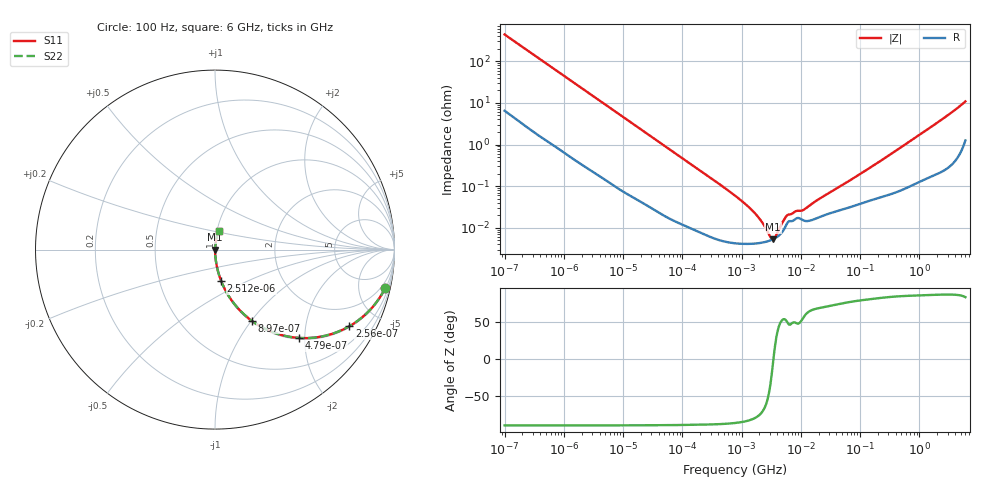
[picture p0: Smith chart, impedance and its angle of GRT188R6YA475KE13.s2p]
!Murata Part Number: GRT188R6YA475KE13
!These Parameters are Measured in Series Mode Connection
!Data Generated on Jun 19, 2026
!  o--ll--o
!Port1  Port2
!  o------o
!Operation Temp=25[degC], DC Bias Voltage=0[V]
!Freq. Start=100[Hz] Stop=6[GHz] 401[Steps]
# Hz S RI R 50
!Freq.(Hz) S11(Real) S11(Imag) S21(Real) S21(Imag) S12(Real) S12(Imag) S22(Real) S22(Imag)
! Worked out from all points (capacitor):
!   401 points, 100 Hz to 6 GHz, reference 50 ohm
!   read as one part in series: C = 3.6 uF near 109 Hz
!   lowest |Z| = 5.31 mohm at 3.394 MHz (marker M1)
!   series resonance near 3.45 MHz, so ESL is about 590 pH
!   S11 on the Smith chart (normalised r, x): 100 Hz: 1.13, -8.81; 256 Hz: 1.05, -3.47; 479 Hz: 1.03, -1.86; 897 Hz: 1.01, -1.00; 2.512 kHz: 1.01, -0.36; 6 GHz: 1.03, +0.22
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100  0.9481 -0.2145  0.0519 0.2145  0.0519 0.2145  0.9481 -0.2145
164  0.8762 -0.3222  0.1238 0.3222  0.1238 0.3222  0.8762 -0.3222
256  0.7478 -0.4274  0.2522 0.4274  0.2522 0.4274  0.7478 -0.4274
479  0.4653 -0.4919  0.5347 0.4919  0.5347 0.4919  0.4653 -0.4919
897  0.2039 -0.3958  0.7961 0.3958  0.7961 0.3958  0.2039 -0.3958
2008  0.0511 -0.213  0.9489 0.213  0.9489 0.213  0.0511 -0.213
2512  0.0339 -0.1738  0.9661 0.1738  0.9661 0.1738  0.0339 -0.1738
7695  0.00446 -0.0592  0.9955 0.0592  0.9955 0.0592  0.00446 -0.0592
40335  0.000362 -0.0115  0.9996 0.0115  0.9996 0.0115  0.000362 -0.0115
774597  4.26e-05 -0.00059  1 0.00059  1 0.00059  4.26e-05 -0.00059
1516199  4.13e-05 -0.000257  1 0.000257  1 0.000257  4.13e-05 -0.000257
2481164  4.54e-05 -9.48e-05  1 9.48e-05  1 9.48e-05  4.54e-05 -9.48e-05
2713602  4.7e-05 -6.87e-05  1 6.87e-05  1 6.87e-05  4.7e-05 -6.87e-05
3394479  5.29e-05 -4.6e-06  0.9999 4.6e-06  0.9999 4.6e-06  5.29e-05 -4.6e-06
4246196  6.46e-05 6.14e-05  0.9999 -6.14e-05  0.9999 -6.14e-05  6.46e-05 6.14e-05
6075234  0.000137 0.000153  0.9999 -0.000153  0.9999 -0.000153  0.000137 0.000153
8311524  0.000166 0.000188  0.9998 -0.000188  0.9998 -0.000188  0.000166 0.000188
1.087309e7  0.000152 0.000217  0.9998 -0.000217  0.9998 -0.000217  0.000152 0.000217
1.555665e7  0.000154 0.000348  0.9998 -0.000348  0.9998 -0.000348  0.000154 0.000348
3.124326e8  0.000655 0.00553  0.9993 -0.00553  0.9993 -0.00553  0.000655 0.00553
1.95892e9  0.00297 0.0324  0.997 -0.0324  0.997 -0.0324  0.00297 0.0324
6e9  0.0234 0.104  0.9766 -0.104  0.9766 -0.104  0.0234 0.104
